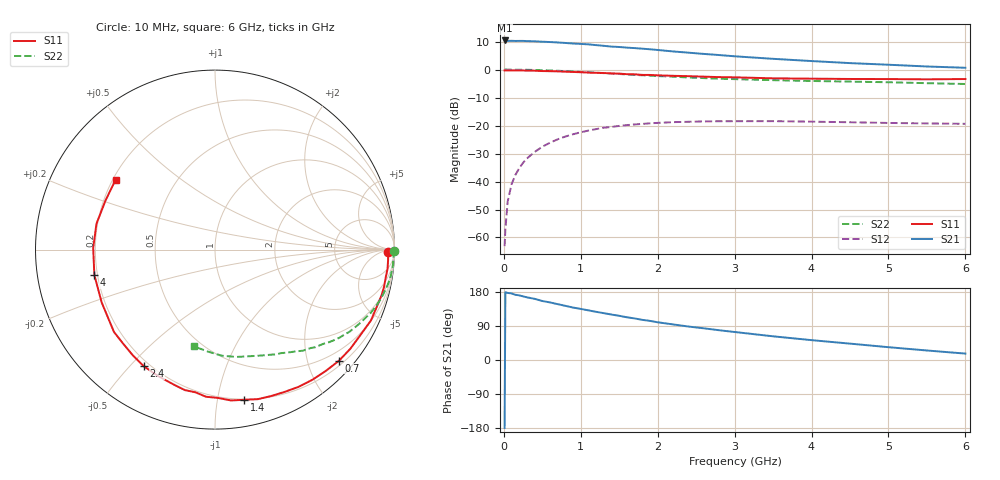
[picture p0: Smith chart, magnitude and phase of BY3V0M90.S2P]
! SIEMENS Small Signal Semiconductors
! BFY420
! Si NPN RF SIEGET Grounded Emitter Transistor in MICRO-X
! VCE = 3 V  IC = 0.9 mA
! Common Emitter S-Parameters:  October  1996
# GHz  S  MA  R  50
!  f  S11  S21  S12  S22
! GHz  MAG  ANG  MAG  ANG  MAG  ANG  MAG  ANG
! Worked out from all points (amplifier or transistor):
!   36 points, 10 MHz to 6 GHz, reference 50 ohm
!   highest |S21| = 10.4 dB at 10 MHz (marker M1)
!   |S21| within 3 dB of that: start of sweep to 1.829 GHz
!   unconditionally stable (mu >= 1): 4.579 GHz to end of sweep
!   at 250 MHz: K = 0.03, MSG = 21.8 dB, |S12| = -33.3 dB
!   at 1.4 GHz: K = 0.18, MSG = 14.4 dB, |S12| = -20.5 dB
!   at 6 GHz: K = 1.35, MAG = 6.5 dB, |S12| = -19.4 dB
!   S11 on the Smith chart (normalised r, x): 10 MHz: 49, -19; 700 MHz: 0.29, -2.59; 1.4 GHz: 0.20, -1.20; 2.4 GHz: 0.18, -0.55; 4 GHz: 0.19, -0.10; 6 GHz: 0.21, +0.30
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0.01  0.9654 -0.8  3.308 -179.4  0.0007 119.8  0.9992 -0.3
0.02  0.9641 -1.2  3.296 178.7  0.0014 93.2  0.9999 -0.6
0.05  0.9662 -3.2  3.251 177.0  0.0044 86.6  0.9972 -1.4
0.1  0.9672 -6.4  3.26 175.7  0.0089 87.1  0.9941 -2.9
0.15  0.9637 -9.2  3.24 172.1  0.0131 84.0  0.995 -4.3
0.2  0.9645 -12.3  3.248 170.6  0.0173 82.7  0.9947 -5.6
0.25  0.9624 -15.2  3.248 167.9  0.0216 80.4  0.9911 -7.1
0.4  0.9544 -24.4  3.196 161.4  0.0337 75.2  0.983 -11.3
0.5  0.9398 -30.4  3.141 155.7  0.0418 72.0  0.9727 -14.1
0.7  0.9278 -41.8  3.048 147.4  0.0568 64.9  0.9511 -19.3
0.9  0.9058 -53.2  2.919 138.4  0.0699 57.7  0.9214 -24.3
1.1  0.8825 -64.0  2.818 131.0  0.0814 51.8  0.8926 -29.0
1.4  0.8527 -78.9  2.569 119.9  0.0943 43.3  0.8495 -35.3
1.8  0.8026 -97.8  2.358 105.9  0.1069 33.3  0.7899 -42.5
2.2  0.7727 -114.2  2.106 93.9  0.1149 25.0  0.7461 -49.0
2.4  0.7615 -121.3  2.002 88.3  0.1167 21.9  0.7209 -52.0
2.8  0.7325 -134.3  1.815 78.5  0.1193 15.7  0.6851 -57.3
3.5  0.6966 -155.0  1.554 62.5  0.1197 7.8  0.6463 -65.8
4  0.6869 -168.1  1.418 52.4  0.1173 3.9  0.6245 -72.1
4.5  0.6787 179.3  1.303 43.2  0.1144 0.9  0.6098 -78.7
5.5  0.6685 155.7  1.134 25.1  0.109 -0.8  0.5705 -93.6
6  0.6771 144.8  1.076 16.9  0.1073 0.1  0.5521 -102.1
